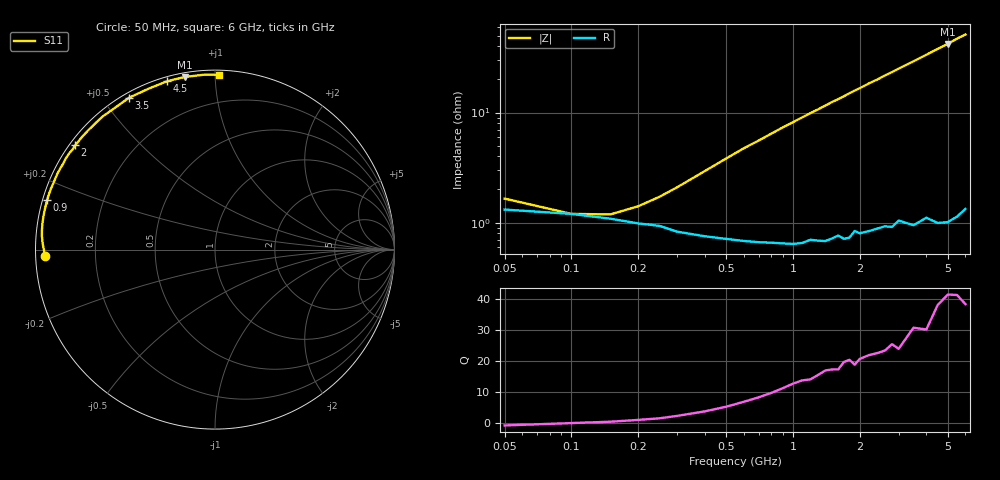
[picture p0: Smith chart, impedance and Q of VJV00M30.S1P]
! Infineon Technologies  Discrete & RF Semiconductors
! BB 914
! Si Tuning Diode in SOT23
! VR =
! S-Parameters:  July  1999
# GHz  S  MA  R  50
!  f  S11
! GHz  MAG  ANG
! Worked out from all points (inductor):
!   34 points, 50 MHz to 6 GHz, reference 50 ohm
!   read as one part to ground: L = 1.22 nH near 400 MHz
!   highest Q = 41.3 at 5 GHz (marker M1), where L = 1.34 nH
!   S11 on the Smith chart (normalised r, x): 50 MHz: 0.03, -0.02; 900 MHz: 0.01, +0.15; 2 GHz: 0.02, +0.33; 3.5 GHz: 0.02, +0.58; 4.5 GHz: 0.02, +0.76; 6 GHz: 0.03, +1.02
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0.05  0.9488 -177.7
0.1  0.9531 -180.0
0.2  0.9614 177.7
0.3  0.9675 175.6
0.4  0.9705 173.5
0.6  0.9734 169.3
0.8  0.9745 165.4
0.9  0.975 163.4
1.1  0.975 159.6
1.3  0.9741 155.9
1.4  0.9745 154.0
1.5  0.9734 152.1
1.6  0.9719 150.4
1.7  0.9739 148.6
1.8  0.9735 146.7
1.9  0.9699 144.9
2  0.9716 143.3
2.2  0.9709 139.7
2.4  0.97 136.6
2.6  0.9693 133.1
2.8  0.9704 130.1
3  0.9671 126.8
3.5  0.9721 119.5
4  0.9699 112.4
4.5  0.9751 105.8
5  0.9765 100.0
5.5  0.9761 93.7
6  0.9743 88.7
